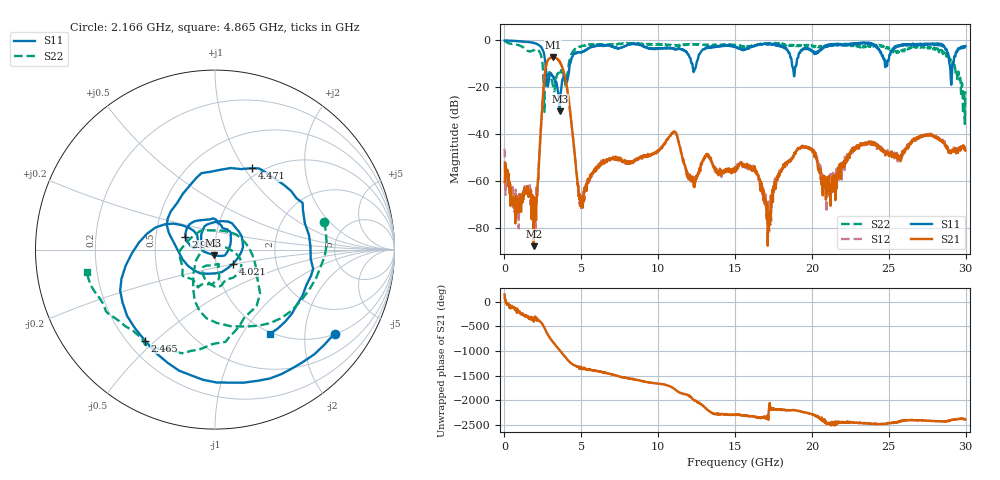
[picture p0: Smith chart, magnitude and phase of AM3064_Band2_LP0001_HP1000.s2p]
# Hz S DB R 50.0
!freq dBS11 angS11 dBS21 angS21 dBS12 angS12 dBS22 angS22
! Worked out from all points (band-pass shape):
!   1600 points, 10 MHz to 29.98 GHz, reference 50 ohm
!   highest |S21| = -7.07 dB at 3.159 GHz (marker M1); lowest = -87.9 dB at 1.903 GHz (marker M2)
!   |S21| within 3 dB of the highest: 2.734 GHz to 3.661 GHz (927.2 MHz wide, 29 % of centre)
!   lowest |S11| = -30.3 dB at 3.59 GHz (marker M3), VSWR 1.06, Z = 49.1 - j2.87 ohm
!   |S11| at or under -10 dB: 2.671 GHz to 4.267 GHz (1.596 GHz wide, 46 % of centre); 18.7 GHz to 19 GHz (298.1 MHz wide, 1.58 % of centre); 28.95 GHz to 29.2 GHz (256.4 MHz wide, 0.882 % of centre)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
!   |S22| runs from -35.7 to -0.2 dB; largest |S21 - S12| = 0.015
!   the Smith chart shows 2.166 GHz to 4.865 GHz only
!   S11 on the Smith chart (normalised r, x): 2.166 GHz: 1.02, -2.83; 2.465 GHz: 0.27, -0.46; 2.934 GHz: 0.71, +0.11; 4.021 GHz: 1.21, -0.19; 4.471 GHz: 0.90, +1.09; 4.865 GHz: 0.98, -1.34
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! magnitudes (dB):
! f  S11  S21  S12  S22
! 10 MHz  0.0  -60.6  -46.3  -0.2
! 1.903 GHz  -1.0  -87.9  -67.9  -4.2
! 2.166 GHz  -1.8  -61.1  -61.7  -4.0
! 2.465 GHz  -3.9  -27.5  -27.5  -9.1
! 2.934 GHz  -14.9  -7.7  -7.7  -13.6
! 3.159 GHz  -15.3  -7.1  -7.3  -20.0
! 3.59 GHz  -30.3  -9.0  -9.2  -12.8
! 4.021 GHz  -17.8  -18.5  -18.5  -17.8
! 4.471 GHz  -6.1  -42.4  -42.0  -4.4
! 4.865 GHz  -5.0  -67.7  -67.2  -2.8
! 5.015 GHz  -5.2  -70.7  -70.6  -2.6
! 10 GHz  -3.5  -47.2  -47.1  -1.7
! 15 GHz  -2.7  -56.3  -55.4  -1.8
! 16.37 GHz  -2.0  -56.9  -55.8  -2.1
! 17.16 GHz  -1.6  -80.4  -68.8  -1.4
! 18.08 GHz  -2.3  -54.7  -54.1  -1.6
! 19.99 GHz  -4.4  -46.9  -46.5  -2.1
! 21.17 GHz  -1.8  -66.9  -64.3  -1.7
! 23.05 GHz  -1.1  -46.3  -44.9  -2.5
! 25 GHz  -8.3  -49.0  -48.9  -3.0
! 28.56 GHz  -2.5  -43.5  -43.4  -4.8
! 29.98 GHz  -2.4  -47.1  -47.0  -21.8
